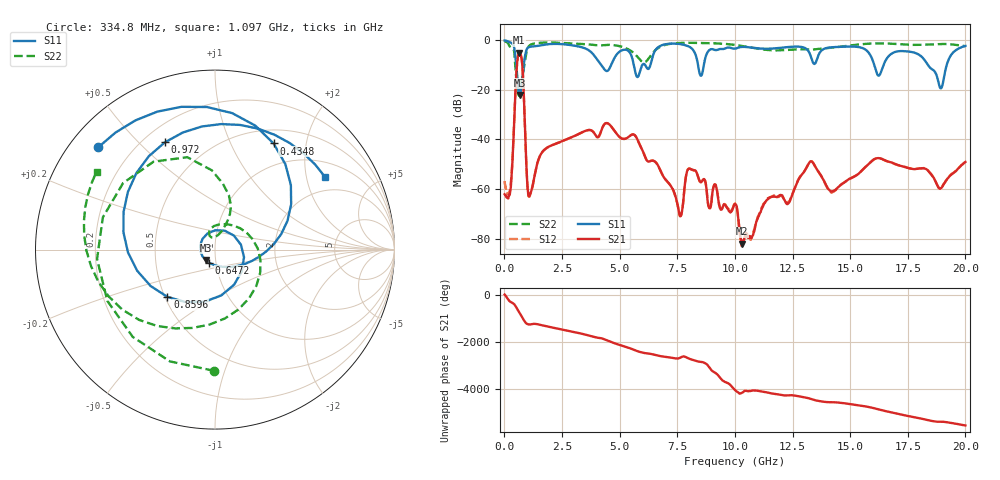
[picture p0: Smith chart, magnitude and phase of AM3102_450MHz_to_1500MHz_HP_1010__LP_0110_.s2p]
!Agilent Technologies,E8364B,MY43040894,A.07.50.67
!Agilent E8364B: A.07.50.67
!Date: Thursday, January 11, 2018 06:11:37
!Correction: S11(Full 2 Port(1,2))
!S21(Full 2 Port(1,2))
!S12(Full 2 Port(1,2))
!S22(Full 2 Port(1,2))
!S2P File: Measurements: S11, S21, S12, S22:
# Hz S  dB  R 50
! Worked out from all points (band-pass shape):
!   1601 points, 10 MHz to 20 GHz, reference 50 ohm
!   highest |S21| = -5.01 dB at 647.2 MHz (marker M1); lowest = -82.0 dB at 10.3 GHz (marker M2)
!   |S21| within 3 dB of the highest: 565.9 MHz to 755.7 MHz (189.7 MHz wide, 28.7 % of centre)
!   lowest |S11| = -22.1 dB at 659.7 MHz (marker M3), VSWR 1.17, Z = 44.7 - j5.23 ohm
!   |S11| at or under -10 dB: 4.201 GHz to 4.629 GHz (427.8 MHz wide, 9.69 % of centre); 16.05 GHz to 16.45 GHz (399.7 MHz wide, 2.46 % of centre); 18.38 GHz to 19.19 GHz (810.9 MHz wide, 4.32 % of centre)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
!   |S22| runs from -23.3 to -0.4 dB; largest |S21 - S12| = 0.00078
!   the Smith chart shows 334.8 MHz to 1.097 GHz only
!   S11 on the Smith chart (normalised r, x): 334.8 MHz: 0.08, +0.37; 434.8 MHz: 0.68, +1.47; 647.2 MHz: 0.93, -0.14; 859.6 MHz: 0.51, -0.32; 972 MHz: 0.28, +0.60; 1.097 GHz: 1.49, +2.60
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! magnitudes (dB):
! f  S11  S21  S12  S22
! 10 MHz  -0.1  -62.1  -56.8  -0.4
! 334.8 MHz  -1.3  -51.5  -50.9  -3.4
! 434.8 MHz  -3.4  -30.0  -29.9  -5.4
! 647.2 MHz  -21.9  -5.0  -5.0  -23.0
! 659.7 MHz  -22.1  -5.0  -5.0  -21.9
! 859.6 MHz  -8.5  -26.2  -26.1  -10.3
! 972 MHz  -3.6  -54.0  -54.2  -4.2
! 1.097 GHz  -2.7  -62.5  -62.9  -2.0
! 1.684 GHz  -1.9  -44.6  -44.6  -0.9
! 3.346 GHz  -2.8  -37.2  -37.2  -1.5
! 5.782 GHz  -14.8  -40.2  -40.2  -6.7
! 6.682 GHz  -2.7  -50.8  -50.9  -3.1
! 7.619 GHz  -1.5  -71.0  -70.7  -1.1
! 8.043 GHz  -2.7  -51.7  -51.8  -1.0
! 8.531 GHz  -14.3  -57.3  -57.4  -1.1
! 10.01 GHz  -3.4  -66.1  -65.8  -1.9
! 10.3 GHz  -2.7  -82.0  -82.9  -2.3
! 13.34 GHz  -7.8  -48.9  -48.9  -3.8
! 14.22 GHz  -2.8  -61.0  -61.4  -3.0
! 16.68 GHz  -6.3  -48.9  -48.9  -1.3
! 18.94 GHz  -19.4  -59.7  -59.5  -1.5
! 20 GHz  -2.3  -49.1  -49.2  -2.4
